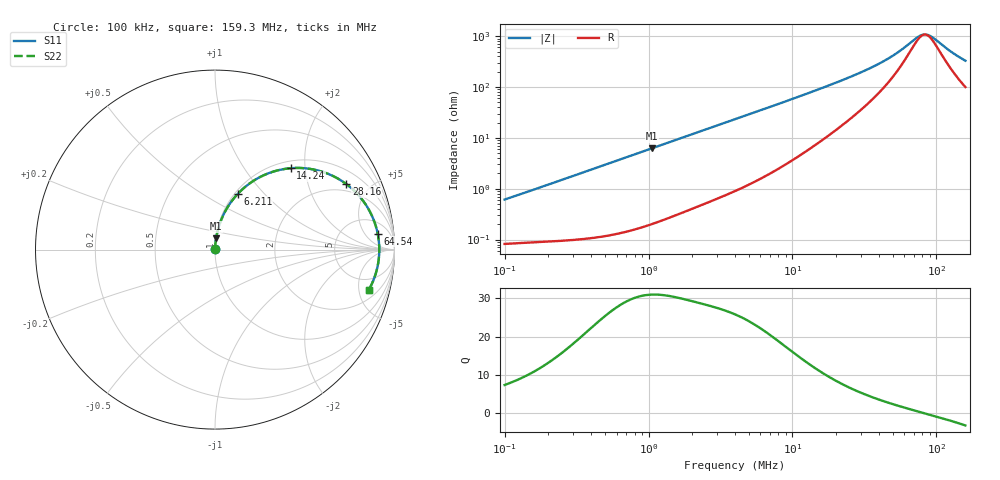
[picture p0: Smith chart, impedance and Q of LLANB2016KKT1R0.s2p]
! LLANB2016KKT1R0  S-PARAMETER MODEL  ( General Type )
! Model Generated by TAIYO YUDEN Corporation (http://www.ty-top.com)
! Version 3.0
! TAIYO YUDEN Control No. 160323NG38SB-FKC
! Copyright(c) 2012 TAIYO YUDEN CO.,LTD. All Rights Reserved.
! Product Description (link to TY-COMPAS)
! https://ds.yuden.co.jp/TYCOMPAS/or/detail?pn=LLANB2016KKT1R0M&u=M
! Products Name : Inductors
! Characteristics :
!  Inductance : 1.0 uH , SRF(min) : -Hz , DC Resistance(max) : 0.075 Ohm
!  Rated Current : Saturation :2200 mA , Temp Rise : 2200 mA (40 degC)
!  Case Size : 2.0 x 1.6 / 0.079 x 0.063 [mm/inch] , Thickness : 1 / 0.039 [mm/inch]
!  (Conditions: Temperature = 25 degC , DC Bias Current/Voltage = 0A / 0V)
! External Node Assignments :
!  1  o---GGG---o  2
! GND o---------o GND
! Frequency Range : 0.1MHz  -  159.254811MHz  [ 402 STEP ]
# MHz S RI R 50
! Freq[MHz].  S11 Real  S11 Imag  S21 Real  S21 Imag  S12 Real  S12 Imag  S22 Real  S22 Imag
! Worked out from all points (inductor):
!   401 points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, 100 kHz to 159.3 MHz, reference 50 ohm
!   read as one part in series: L = 960 nH near 103.8 kHz
!   highest Q = 30.9 at 1.058 MHz (marker M1), where L = 940 nH
!   self-resonance near 83.33 MHz
!   S11 on the Smith chart (normalised r, x): 100 kHz: 1.00, +0.01; 6.211 MHz: 1.03, +0.72; 14.24 MHz: 1.14, +1.68; 28.16 MHz: 1.61, +3.56; 64.54 MHz: 10, +11; 159.3 MHz: 3.00, -6.27
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0.1  0.000858 0.00606  0.9991 -0.00606  0.9991 -0.00606  0.000858 0.00606
0.343835  0.00144 0.0204  0.9986 -0.0204  0.9986 -0.0204  0.00144 0.0204
1.058448  0.00589 0.062  0.9941 -0.062  0.9941 -0.062  0.00589 0.062
1.182227  0.00706 0.0691  0.9929 -0.0691  0.9929 -0.0691  0.00706 0.0691
2.295564  0.0221 0.1306  0.9779 -0.1306  0.9779 -0.1306  0.0221 0.1306
4.064915  0.0605 0.2197  0.9395 -0.2197  0.9395 -0.2197  0.0605 0.2197
6.211147  0.126 0.3097  0.874 -0.3097  0.874 -0.3097  0.126 0.3097
9.147063  0.2342 0.3953  0.7658 -0.3953  0.7658 -0.3953  0.2342 0.3953
13.72135  0.4038 0.4517  0.5962 -0.4517  0.5962 -0.4517  0.4038 0.4517
14.23663  0.4213 0.4535  0.5787 -0.4535  0.5787 -0.4535  0.4213 0.4535
19.83816  0.5821 0.4384  0.4179 -0.4384  0.4179 -0.4384  0.5821 0.4384
28.15793  0.7315 0.3652  0.2685 -0.3652  0.2685 -0.3652  0.7315 0.3652
37.1261  0.8183 0.2806  0.1817 -0.2806  0.1817 -0.2806  0.8183 0.2806
47.17884  0.8694 0.199  0.1306 -0.199  0.1306 -0.199  0.8694 0.199
54.67504  0.8907 0.1475  0.1093 -0.1475  0.1093 -0.1475  0.8907 0.1475
64.54108  0.9064 0.0893  0.0936 -0.0893  0.0936 -0.0893  0.9064 0.0893
77.60479  0.9146 0.0249  0.0854 -0.0249  0.0854 -0.0249  0.9146 0.0249
82.01707  0.9153 0.00555  0.0847 -0.00555  0.0847 -0.00555  0.9153 0.00555
86.6802  0.9152 -0.0138  0.0848 0.0138  0.0848 0.0138  0.9152 -0.0138
95.04868  0.9131 -0.046  0.0869 0.046  0.0869 0.046  0.9131 -0.046
132.4464  0.8858 -0.1624  0.1142 0.1624  0.1142 0.1624  0.8858 -0.1624
159.2548  0.8556 -0.2268  0.1444 0.2268  0.1444 0.2268  0.8556 -0.2268
